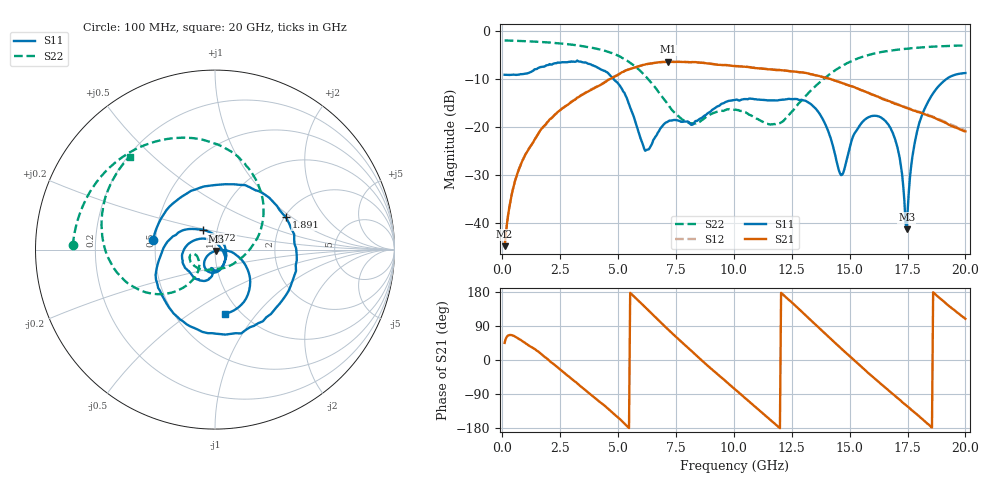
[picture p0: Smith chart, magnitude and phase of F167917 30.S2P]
!  2-Port S-parameters saved by WinCal
! VAR MeasName=S-Parameters (CALIBRATED_DATA) read from VNA (N5242A)
! VAR MeasDate=2016-11-22 9:01:12
! VAR NAME=F167917 30
! VAR FILENAME=F167917 30.S2P
! VAR DATE=2016-11-22 9:01:12
! VAR PHYS_PORTS=1,2
# Hz S DB R 50
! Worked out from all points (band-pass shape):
!   401 points, 100 MHz to 20 GHz, reference 50 ohm
!   highest |S21| = -6.47 dB at 7.165 GHz (marker M1); lowest = -44.9 dB at 100 MHz (marker M2)
!   |S21| within 3 dB of the highest: 4.885 GHz to 13.71 GHz (8.822 GHz wide, 94.9 % of centre)
!   lowest |S11| = -41.3 dB at 17.46 GHz (marker M3), VSWR 1.02, Z = 50.5 - j0.733 ohm
!   |S11| at or under -10 dB: 4.79 GHz to 19.2 GHz (14.41 GHz wide, 120 % of centre)
!   |S22| runs from -19.5 to -2.0 dB; largest |S21 - S12| = 0.0046
!   S11 on the Smith chart (normalised r, x): 100 MHz: 0.49, +0.06; 1.891 GHz: 2.03, +0.91; 5.672 GHz: 0.86, +0.19; 20 GHz: 0.85, -0.70
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1e8  -9.17 171.3  -44.87 45.3  -44.81 45.7  -2.03 178.3
6.97e8  -9.16 120.5  -29.12 56.3  -29.07 56.2  -2.12 168.7
1.891e9  -7.24 24.6  -19.43 5.6  -19.43 5.5  -2.41 149.5
2.53775e9  -6.60 -26.0  -16.39 -27.2  -16.38 -27.1  -2.66 138.2
3.43325e9  -6.52 -86.1  -13.40 -71.9  -13.34 -71.8  -3.19 120.9
4.52775e9  -8.65 -152.7  -10.40 -126.1  -10.35 -126.4  -4.33 94.3
5.672e9  -17.81 121.1  -7.73 168.7  -7.73 168.4  -7.19 56.7
6.21925e9  -24.85 29.9  -6.96 136.3  -6.97 136.1  -9.65 35.1
6.7665e9  -20.90 -54.7  -6.56 103.8  -6.57 103.7  -12.90 10.7
7.1645e9  -18.87 -80.3  -6.47 80.3  -6.47 80.4  -15.43 -9.8
8.50775e9  -18.41 -95.2  -6.64 4.8  -6.60 4.9  -19.00 -101.0
1.005e10  -14.42 -115.4  -7.35 -77.3  -7.34 -77.2  -16.47 -158.9
1.179125e10  -14.50 -139.9  -8.16 -169.4  -8.12 -169.5  -19.46 -150.9
1.338325e10  -15.52 176.6  -9.08 101.5  -9.10 101.6  -12.17 -127.9
1.4627e10  -30.06 48.2  -10.80 30.9  -10.78 31.1  -7.47 -144.5
1.5622e10  -18.65 -76.1  -12.57 -24.0  -12.58 -23.6  -5.33 -163.0
1.67165e10  -19.90 -126.9  -14.67 -82.0  -14.67 -81.5  -4.17 177.8
1.71145e10  -25.40 -140.8  -15.47 -102.2  -15.37 -102.2  -3.93 171.5
1.746275e10  -41.32 -57.8  -16.10 -120.9  -15.98 -120.1  -3.74 166.5
1.7811e10  -23.35 -4.9  -16.68 -138.7  -16.61 -138.2  -3.59 161.5
1.8209e10  -16.59 -19.0  -17.30 -160.0  -17.19 -159.3  -3.43 155.9
2e10  -8.81 -81.6  -20.95 108.6  -20.73 108.7  -3.09 132.6
